FUNCTION_BLOCK "FB_ALE 203"
TITLE =
VERSION : 0.1


VAR
  WaterTemp_A1 : "fb_AnalogIN"; //Water Temperature ALE 203
WaterFlow_A1 : "fb_AnalogIN"; //Water Flowrate ALE 203
WaterTemp_A2 : "fb_AnalogIN"; //Water Temperature ALE 203
WaterFlow_A2 : "fb_AnalogIN"; //Water Flowrate ALE 203
END_VAR
BEGIN
NETWORK
TITLE =
CALL #WaterTemp_A1 (In_V_CAMPO:= PEW 316);
CALL #WaterFlow_A1 (In_V_CAMPO:= PEW 318);
CALL #WaterTemp_A2 (In_V_CAMPO:= PEW 444);
CALL #WaterFlow_A2 (In_V_CAMPO:= PEW 446);

END_FUNCTION_BLOCK

FUNCTION_BLOCK "FB_ARC_DET"
TITLE =
VERSION : 0.1


VAR
 Arc1_A1 : "fb_DI_IN"; //Water Flowrate ALE 203
PwrFail1_A1 : "fb_DI_IN"; // Arc Detector Signal 1
Arc2_A1 : "fb_DI_IN"; //Power Fail in Arc Detector 1
PwrFail2_A1 : "fb_DI_IN"; // Arc Detector Signal 2
Arc3_A1 : "fb_DI_IN"; //Power Fail in Arc Detector 2
PwrFail3_A1 : "fb_DI_IN"; // Arc Detector Signal 3
Arc4_A1 : "fb_DI_IN"; //Power Fail in Arc Detector 3
PwrFail4_A1 : "fb_DI_IN"; // Arc Detector Signal 4
Arc5_A1 : "fb_DI_IN"; //Power Fail in Arc Detector 4
PwrFail5_A1 : "fb_DI_IN"; // Arc Detector Signal 5
Arc6_A1 : "fb_DI_IN"; //Power Fail in Arc Detector 5
PwrFail6_A1 : "fb_DI_IN"; // Arc Detector Signal 6
Arc7_A1 : "fb_DI_IN"; //Power Fail in Arc Detector 6
PwrFail7_A1 : "fb_DI_IN"; // Arc Detector Signal 7
Arc8_A1 : "fb_DI_IN"; //Power Fail in Arc Detector 7
PwrFail8_A1 : "fb_DI_IN"; // Arc Detector Signal 8
Arc1_A2 : "fb_DI_IN"; //Power Fail in Arc Detector 8
PwrFail1_A2 : "fb_DI_IN"; // Arc Detector Signal 1
Arc2_A2 : "fb_DI_IN"; //Power Fail in Arc Detector 1
PwrFail2_A2 : "fb_DI_IN"; // Arc Detector Signal 2
Arc3_A2 : "fb_DI_IN"; //Power Fail in Arc Detector 2
PwrFail3_A2 : "fb_DI_IN"; // Arc Detector Signal 3
Arc4_A2 : "fb_DI_IN"; //Power Fail in Arc Detector 3
PwrFail4_A2 : "fb_DI_IN"; // Arc Detector Signal 4
Arc5_A2 : "fb_DI_IN"; //Power Fail in Arc Detector 4
PwrFail5_A2 : "fb_DI_IN"; // Arc Detector Signal 5
Arc6_A2 : "fb_DI_IN"; //Power Fail in Arc Detector 5
PwrFail6_A2 : "fb_DI_IN"; // Arc Detector Signal 6
Arc7_A2 : "fb_DI_IN"; //Power Fail in Arc Detector 6
PwrFail7_A2 : "fb_DI_IN"; // Arc Detector Signal 7
Arc8_A2 : "fb_DI_IN"; //Power Fail in Arc Detector 7
PwrFail8_A2 : "fb_DI_IN"; // Arc Detector Signal 8
END_VAR
BEGIN
NETWORK
TITLE =
CALL #Arc1_A1 (V_CAMPO:= E 8.1);
CALL #PwrFail1_A1 (V_CAMPO:= E 8.3);
CALL #Arc2_A1 (V_CAMPO:= E 8.5);
CALL #PwrFail2_A1 (V_CAMPO:= E 8.7);
CALL #Arc3_A1 (V_CAMPO:= E 9.1);
CALL #PwrFail3_A1 (V_CAMPO:= E 9.3);
CALL #Arc4_A1 (V_CAMPO:= E 9.5);
CALL #PwrFail4_A1 (V_CAMPO:= E 9.7);
CALL #Arc5_A1 (V_CAMPO:= E 10.3);
CALL #PwrFail5_A1 (V_CAMPO:= E 10.5);
CALL #Arc6_A1 (V_CAMPO:= E 10.7);
CALL #PwrFail6_A1 (V_CAMPO:= E 11.1);
CALL #Arc7_A1 (V_CAMPO:= E 11.3);
CALL #PwrFail7_A1 (V_CAMPO:= E 11.5);
CALL #Arc8_A1 (V_CAMPO:= E 11.7);
CALL #PwrFail8_A1 (V_CAMPO:= E 12.1);
CALL #Arc1_A2 (V_CAMPO:= E 32.1);
CALL #PwrFail1_A2 (V_CAMPO:= E 32.3);
CALL #Arc2_A2 (V_CAMPO:= E 32.5);
CALL #PwrFail2_A2 (V_CAMPO:= E 32.7);
CALL #Arc3_A2 (V_CAMPO:= E 33.1);
CALL #PwrFail3_A2 (V_CAMPO:= E 33.3);
CALL #Arc4_A2 (V_CAMPO:= E 33.5);
CALL #PwrFail4_A2 (V_CAMPO:= E 33.7);
CALL #Arc5_A2 (V_CAMPO:= E 34.3);
CALL #PwrFail5_A2 (V_CAMPO:= E 34.5);
CALL #Arc6_A2 (V_CAMPO:= E 34.7);
CALL #PwrFail6_A2 (V_CAMPO:= E 35.1);
CALL #Arc7_A2 (V_CAMPO:= E 35.3);
CALL #PwrFail7_A2 (V_CAMPO:= E 35.5);
CALL #Arc8_A2 (V_CAMPO:= E 35.7);
CALL #PwrFail8_A2 (V_CAMPO:= E 36.1);

END_FUNCTION_BLOCK

FUNCTION_BLOCK "FB_ARC_GLOB"
TITLE =
VERSION : 0.1


VAR
 Arc_A2 : "fb_AnalogIN"; //Global Arc
Arc : "fb_AnalogIN"; //Global Arc
GlobReset_AC : "fb_DI_OUT"; //Global Arc
GlobTest_AC : "fb_DI_OUT"; //Global Reset
GlobReset_A2 : "fb_DI_OUT"; //Global Test
GlobTest_A2 : "fb_DI_OUT"; //Global Reset
END_VAR
BEGIN
NETWORK
TITLE =
CALL #Arc_A2 (In_V_CAMPO:= PEW 462);
CALL #Arc (In_V_CAMPO:= PEW 334);
CALL #GlobReset_AC (OUT:= A 16.0);
CALL #GlobTest_AC (OUT:= A 16.1);
CALL #GlobReset_A2 (OUT:= A 32.0);
CALL #GlobTest_A2 (OUT:= A 32.1);

END_FUNCTION_BLOCK
FUNCTION_BLOCK "FB_CIRC"
TITLE =
VERSION : 0.1


VAR
 Arc_A2 : "fb_AnalogIN"; //Global Arc
Arc : "fb_AnalogIN"; //Global Arc
GlobReset_AC : "fb_DI_OUT"; //Global Arc
GlobTest_AC : "fb_DI_OUT"; //Global Reset
GlobReset_A2 : "fb_DI_OUT"; //Global Test
GlobTest_A2 : "fb_DI_OUT"; //Global Reset
END_VAR
BEGIN
NETWORK
TITLE =
CALL #Arc_A2 (In_V_CAMPO:= PEW 462);
CALL #Arc (In_V_CAMPO:= PEW 334);
CALL #GlobReset_AC (OUT:= A 16.0);
CALL #GlobTest_AC (OUT:= A 16.1);
CALL #GlobReset_A2 (OUT:= A 32.0);
CALL #GlobTest_A2 (OUT:= A 32.1);

END_FUNCTION_BLOCK
FUNCTION_BLOCK "FB_CPLT"
TITLE = VERSION : 0.1
VAR
WaterRes_AC : "fb_AnalogIN"; //Resistivity
WaterPress_AC : "fb_AnalogIN"; //Pressure Input
WaterTemp_AC : "fb_AnalogIN"; //Temperature Input
END_VAR
BEGIN
NETWORK
TITLE =
CALL #WaterRes_AC (In_V_CAMPO:= PEW 288);
CALL #WaterPress_AC (In_V_CAMPO:= PEW 290);
CALL #WaterTemp_AC (In_V_CAMPO:= PEW 292);
END_FUNCTION_BLOCK
FUNCTION_BLOCK "FB_CSPS"
 TITLE =
 VERSION : 0.1
 VAR
Vread1_1_A1 : "fb_AnalogIN"; //Voltage Monitor 1.1
Vread1_2_A1 : "fb_AnalogIN"; //Voltage Monitor 1.2
Vread1_3_A1 : "fb_AnalogIN"; //Voltage Monitor 1.3
Vread1_4_A1 : "fb_AnalogIN"; //Voltage Monitor 1.4
Vread1_1_A2 : "fb_AnalogIN"; //Voltage Monitor 2.1
Vread1_2_A2 : "fb_AnalogIN"; //Voltage Monitor 2.2
Vread1_3_A2 : "fb_AnalogIN"; //Voltage Monitor 2.3
Vread1_4_A2 : "fb_AnalogIN"; //Voltage Monitor 2.4
END_VAR
BEGIN
NETWORK
TITLE =
CALL #Vread1_1_A1 (In_V_CAMPO:= PEW 352);
CALL #Vread1_2_A1 (In_V_CAMPO:= PEW 354);
CALL #Vread1_3_A1 (In_V_CAMPO:= PEW 356);
CALL #Vread1_4_A1 (In_V_CAMPO:= PEW 358);
CALL #Vread1_1_A2 (In_V_CAMPO:= PEW 480);
CALL #Vread1_2_A2 (In_V_CAMPO:= PEW 482);
CALL #Vread1_3_A2 (In_V_CAMPO:= PEW 484);
CALL #Vread1_4_A2 (In_V_CAMPO:= PEW 486);

END_FUNCTION_BLOCK
FUNCTION_BLOCK "FB_DAMP_ACSI"
TITLE =
VERSION : 0.1 VAR
AirPress_A1 : "fb_AnalogIN"; //TH561 Air Press (RF Input)
AirPress_A2 : "fb_AnalogIN"; //TH561 Air Press (RF Input)
AirFlow_A1 : "fb_DI_IN"; //TH561 Air Press (RF Input)
AirFlow_A2 : "fb_DI_IN"; //TH561 Air Flow-rate (RF Input)

END_VAR BEGIN NETWORK TITLE =
CALL #AirPress_A1 (In_V_CAMPO:= PEW 268);
CALL #AirPress_A2 (In_V_CAMPO:= PEW 396);
CALL #AirFlow_A1 (V_CAMPO:= E 16.4);
CALL #AirFlow_A2 (V_CAMPO:= E 40.4);
END_FUNCTION_BLOCK
 FUNCTION_BLOCK "FB_DAMP_ACSO"
TITLE = VERSION : 0.1
VAR
AirPress_A1 : "fb_AnalogIN"; //TH561 Air Press (RF Output)
AirPress_A2 : "fb_AnalogIN"; //TH561 Air Press (RF Output)
AirFlow_A1 : "fb_DI_IN"; //TH561 Air Press (RF Output)
AirFlow_A2 : "fb_DI_IN"; //TH561 Air Flow-rate (RF Output)
END_VAR
BEGIN
NETWORK
TITLE =
CALL #AirPress_A1 (In_V_CAMPO:= PEW 270);
CALL #AirPress_A2 (In_V_CAMPO:= PEW 398);
CALL #AirFlow_A1 (V_CAMPO:= E 16.6);
CALL #AirFlow_A2 (V_CAMPO:= E 40.6);
END_FUNCTION_BLOCK
 FUNCTION_BLOCK "FB_DAMP_ANOD"
TITLE = VERSION : 0.1
VAR
WaterTemp_A1 : "fb_AnalogIN"; //Anode Temperature Output
WaterFlow_A1 : "fb_AnalogIN"; //Anode water Flowrate
WaterTemp_A2 : "fb_AnalogIN"; //Anode Temperature Output
WaterFlow_A2 : "fb_AnalogIN"; //Anode water Flowrate

END_VAR
BEGIN
NETWORK
TITLE =
CALL #WaterTemp_A1 (In_V_CAMPO:= PEW 304);
CALL #WaterFlow_A1 (In_V_CAMPO:= PEW 306);
CALL #WaterTemp_A2 (In_V_CAMPO:= PEW 432);
CALL #WaterFlow_A2 (In_V_CAMPO:= PEW 434);
END_FUNCTION_BLOCK
 FUNCTION_BLOCK "FB_DAMP_ANPS"
TITLE = VERSION : 0.1
VAR
Vread_A1 : "fb_AnalogIN"; //Voltage Meter
Iread_A1 : "fb_AnalogIN"; //Current Meter
Vanalog_A1 : "fb_AnalogIN"; //Charging voltage waveform
Vread_A2 : "fb_AnalogIN"; //Voltage Meter
Iread_A2 : "fb_AnalogIN"; //Current Meter
Vanalog_A2 : "fb_AnalogIN"; //Charging voltage waveform
Vset_A1 : "fb_AnalogOut"; //Charging voltage waveform
Adwellin_A1 : "fb_AnalogOut"; //Vout Voltage Programming
Vset_A2 : "fb_AnalogOut"; //Auto Dwell
Adwellin_A2 : "fb_AnalogOut"; //Vout Voltage Programming
Enable_A1 : "fb_DI_OUT"; //Auto Dwell
Inhibit_A1 : "fb_DI_OUT"; //ON/OFF
EXT_INTERLOOK_A1 : "fb_DI_OUT"; //INHIBIT
EXT_POWER_A1 : "fb_DI_OUT"; //Ext_InterLook
Enable_A2 : "fb_DI_OUT"; //Ext_Power
Inhibit_A2 : "fb_DI_OUT"; //ON/OFF
EXT_INTERLOOK_A2 : "fb_DI_OUT"; //INHIBIT
EXT_POWER_A2 : "fb_DI_OUT"; //Ext_InterLook
Ready_A1 : "fb_DI_IN"; //Ext_Power
InhibitRtn_A1 : "fb_DI_IN"; //Ready
EndOfChrge_A1 : "fb_DI_IN"; //INHIBIT
ExcRevers_A1 : "fb_DI_IN"; //End of Charge
CoolantWrn_A1 : "fb_DI_IN"; //Excess Reversal
Overvolt_A1 : "fb_DI_IN"; //Coolant Warning
Arc_A1 : "fb_DI_IN"; //Over Voltage
Interlock_A1 : "fb_DI_IN"; //ARC
InFault_A1 : "fb_DI_IN"; //Interlock
AdwellOut_A1 : "fb_DI_IN"; //Input Power Fault
LoadFault_A1 : "fb_DI_IN"; //Auto Dwell Output
CoolantFlt_A1 : "fb_DI_IN"; //Load Fault
PurgePump_A1 : "fb_DI_IN"; //Coolant Fault
Ready_A2 : "fb_DI_IN"; //Purge Pump
InhibitRtn_A2 : "fb_DI_IN"; //Ready
EndOfChrge_A2 : "fb_DI_IN"; //INHIBIT
ExcRevers_A2 : "fb_DI_IN"; //End of Charge
CoolantWrn_A2 : "fb_DI_IN"; //Excess Reversal
Overvolt_A2 : "fb_DI_IN"; //Coolant Warning
Arc_A2 : "fb_DI_IN"; //Over Voltage
Interlock_A2 : "fb_DI_IN"; //ARC
InFault_A2 : "fb_DI_IN"; //Interlock
AdwellOut_A2 : "fb_DI_IN"; //Input Power Fault
LoadFault_A2 : "fb_DI_IN"; //Auto Dwell Output
CoolantFlt_A2 : "fb_DI_IN"; //Load Fault
PurgePump_A2 : "fb_DI_IN"; //Coolant Fault
END_VAR
BEGIN
NETWORK
TITLE =
CALL #Vread_A1 (In_V_CAMPO:= PEW 360);
CALL #Iread_A1 (In_V_CAMPO:= PEW 362);
CALL #Vanalog_A1 (In_V_CAMPO:= PEW 364);
CALL #Vread_A2 (In_V_CAMPO:= PEW 488);
CALL #Iread_A2 (In_V_CAMPO:= PEW 490);
CALL #Vanalog_A2 (In_V_CAMPO:= PEW 492);
CALL #Vset_A1 (PAW_OUT:= PAW 272);
CALL #Adwellin_A1 (PAW_OUT:= PAW 274);
CALL #Vset_A2 (PAW_OUT:= PAW 304);
CALL #Adwellin_A2 (PAW_OUT:= PAW 306);
CALL #Enable_A1 (OUT:= A 24.0);
CALL #Inhibit_A1 (OUT:= A 24.1);
CALL #EXT_INTERLOOK_A1 (OUT:= A 24.2);
CALL #EXT_POWER_A1 (OUT:= A 24.3);
CALL #Enable_A2 (OUT:= A 36.0);
CALL #Inhibit_A2 (OUT:= A 36.1);
CALL #EXT_INTERLOOK_A2 (OUT:= A 36.2);
CALL #EXT_POWER_A2 (OUT:= A 36.3);
CALL #Ready_A1 (V_CAMPO:= E 12.3);
CALL #InhibitRtn_A1 (V_CAMPO:= E 12.5);
CALL #EndOfChrge_A1 (V_CAMPO:= E 12.7);
CALL #ExcRevers_A1 (V_CAMPO:= E 13.1);
CALL #CoolantWrn_A1 (V_CAMPO:= E 13.3);
CALL #Overvolt_A1 (V_CAMPO:= E 13.5);
CALL #Arc_A1 (V_CAMPO:= E 13.7);
CALL #Interlock_A1 (V_CAMPO:= E 14.1);
CALL #InFault_A1 (V_CAMPO:= E 14.5);
CALL #AdwellOut_A1 (V_CAMPO:= E 14.7);
CALL #LoadFault_A1 (V_CAMPO:= E 15.1);
CALL #CoolantFlt_A1 (V_CAMPO:= E 15.3);
CALL #PurgePump_A1 (V_CAMPO:= E 15.5);
CALL #Ready_A2 (V_CAMPO:= E 36.3);
CALL #InhibitRtn_A2 (V_CAMPO:= E 36.5);
CALL #EndOfChrge_A2 (V_CAMPO:= E 36.7);
CALL #ExcRevers_A2 (V_CAMPO:= E 37.1);
CALL #CoolantWrn_A2 (V_CAMPO:= E 37.3);
CALL #Overvolt_A2 (V_CAMPO:= E 37.5);
CALL #Arc_A2 (V_CAMPO:= E 37.7);
CALL #Interlock_A2 (V_CAMPO:= E 38.1);
CALL #InFault_A2 (V_CAMPO:= E 38.5);
CALL #AdwellOut_A2 (V_CAMPO:= E 38.7);
CALL #LoadFault_A2 (V_CAMPO:= E 39.1);
CALL #CoolantFlt_A2 (V_CAMPO:= E 39.3);
CALL #PurgePump_A2 (V_CAMPO:= E 39.5);
END_FUNCTION_BLOCK
 FUNCTION_BLOCK "FB_DAMP_CAV"
TITLE = VERSION : 0.1
VAR
State_A1 : "fb_DI_IN"; //Purge Pump
State_A2 : "fb_DI_IN"; //Driver Amplifier Cavity: Open\Closed
END_VAR
BEGIN
NETWORK
TITLE =
CALL #State_A1 (V_CAMPO:= E 10.4);
CALL #State_A2 (V_CAMPO:= E 34.4);
END_FUNCTION_BLOCK

 FUNCTION_BLOCK "FB_DAMP_CGPS"
TITLE = VERSION : 0.1
VAR
Iread_A1 : "fb_AnalogIN"; //Curret Monitor
Vread_A1 : "fb_AnalogIN"; //Voltage Monitor
Status_A1 : "fb_AnalogIN"; //Power Supply OK Signal
Iread_A2 : "fb_AnalogIN"; //Curret Monitor
Vread_A2 : "fb_AnalogIN"; //Voltage Monitor
Status_A2 : "fb_AnalogIN"; //Power Supply OK Signal
Vset_A1 : "fb_AnalogOut"; //Power Supply OK Signal
Vset_A2 : "fb_AnalogOut"; //Vout Voltage Programming
Enable_A1 : "fb_DI_OUT"; //Vout Voltage Programming
Activate_A1 : "fb_DI_OUT"; //Enable/Disable
Enable_A2 : "fb_DI_OUT"; //ON/OFF
Activate_A2 : "fb_DI_OUT"; //Enable/Disable
END_VAR
BEGIN
NETWORK
TITLE =
CALL #Iread_A1 (In_V_CAMPO:= PEW 262);
CALL #Vread_A1 (In_V_CAMPO:= PEW 264);
CALL #Status_A1 (In_V_CAMPO:= PEW 266);
CALL #Iread_A2 (In_V_CAMPO:= PEW 390);
CALL #Vread_A2 (In_V_CAMPO:= PEW 392);
CALL #Status_A2 (In_V_CAMPO:= PEW 394);
CALL #Vset_A1 (PAW_OUT:= PAW 258);
CALL #Vset_A2 (PAW_OUT:= PAW 290);
CALL #Enable_A1 (OUT:= A 16.4);
CALL #Activate_A1 (OUT:= A 16.5);
CALL #Enable_A2 (OUT:= A 32.4);
CALL #Activate_A2 (OUT:= A 32.5);
END_FUNCTION_BLOCK
 FUNCTION_BLOCK "FB_DAMP_FPS"
TITLE = VERSION : 0.1
VAR
Iread_A1 : "fb_AnalogIN"; //Curret Monitor
Vread_A1 : "fb_AnalogIN"; //Voltage Monitor
Status_A1 : "fb_AnalogIN"; //Power Supply OK Signal
Iread_A2 : "fb_AnalogIN"; //Curret Monitor
Vread_A2 : "fb_AnalogIN"; //Voltage Monitor
Status_A2 : "fb_AnalogIN"; //Power Supply OK Signal
Vset_A1 : "fb_AnalogOut"; //Power Supply OK Signal
Vset_A2 : "fb_AnalogOut"; //Vout Voltage Programming
Enable_A1 : "fb_DI_OUT"; //Vout Voltage Programming
Activate_A1 : "fb_DI_OUT"; //Enable/Disable
Enable_A2 : "fb_DI_OUT"; //ON/OFF
Activate_A2 : "fb_DI_OUT"; //Enable/Disable
END_VAR
BEGIN
NETWORK
TITLE =
CALL #Iread_A1 (In_V_CAMPO:= PEW 256);
CALL #Vread_A1 (In_V_CAMPO:= PEW 258);
CALL #Status_A1 (In_V_CAMPO:= PEW 260);
CALL #Iread_A2 (In_V_CAMPO:= PEW 384);
CALL #Vread_A2 (In_V_CAMPO:= PEW 386);
CALL #Status_A2 (In_V_CAMPO:= PEW 388);
CALL #Vset_A1 (PAW_OUT:= PAW 256);
CALL #Vset_A2 (PAW_OUT:= PAW 288);
CALL #Enable_A1 (OUT:= A 16.2);
CALL #Activate_A1 (OUT:= A 16.3);
CALL #Enable_A2 (OUT:= A 32.2);
CALL #Activate_A2 (OUT:= A 32.3);
END_FUNCTION_BLOCK
 FUNCTION_BLOCK "FB_DAMP_SGPS"
TITLE = VERSION : 0.1
VAR
Iread_A1 : "fb_AnalogIN"; //Curret Monitor
Vread_A1 : "fb_AnalogIN"; //Voltage Monitor
Status_A1 : "fb_AnalogIN"; //Power Supply OK Signal
Iread_A2 : "fb_AnalogIN"; //Curret Monitor
Vread_A2 : "fb_AnalogIN"; //Voltage Monitor
Status_A2 : "fb_AnalogIN"; //Power Supply OK Signal
Vset_A1 : "fb_AnalogOut"; //Power Supply OK Signal
Vset_A2 : "fb_AnalogOut"; //Vout Voltage Programming
Enable_A1 : "fb_DI_OUT"; //Vout Voltage Programming
Activate_A1 : "fb_DI_OUT"; //Enable/Disable
Enable_A2 : "fb_DI_OUT"; //ON/OFF
Activate_A2 : "fb_DI_OUT"; //Enable/Disable
END_VAR
BEGIN
NETWORK
TITLE =
CALL #Iread_A1 (In_V_CAMPO:= PEW 272);
CALL #Vread_A1 (In_V_CAMPO:= PEW 274);
CALL #Status_A1 (In_V_CAMPO:= PEW 276);
CALL #Iread_A2 (In_V_CAMPO:= PEW 400);
CALL #Vread_A2 (In_V_CAMPO:= PEW 402);
CALL #Status_A2 (In_V_CAMPO:= PEW 404);
CALL #Vset_A1 (PAW_OUT:= PAW 260);
CALL #Vset_A2 (PAW_OUT:= PAW 292);
CALL #Enable_A1 (OUT:= A 16.6);
CALL #Activate_A1 (OUT:= A 16.7);
CALL #Enable_A2 (OUT:= A 32.6);
CALL #Activate_A2 (OUT:= A 32.7);
END_FUNCTION_BLOCK
 FUNCTION_BLOCK "FB_FAMP_ACS"
TITLE = VERSION : 0.1
VAR
AirPress_A2 : "fb_AnalogIN"; //TH781 Air Press
AirPress_A1 : "fb_AnalogIN"; //TH781 Air Press
AirFlow_A1 : "fb_DI_IN"; //TH781 Air Press
AirFlow_A2 : "fb_DI_IN"; //TH781 Air Flow Rate

END_VAR
BEGIN
NETWORK
TITLE =
CALL #AirPress_A2 (In_V_CAMPO:= PEW 460);
CALL #AirPress_A1 (In_V_CAMPO:= PEW 332);
CALL #AirFlow_A1 (V_CAMPO:= E 17.0);
CALL #AirFlow_A2 (V_CAMPO:= E 41.0);

END_FUNCTION_BLOCK
 FUNCTION_BLOCK "FB_FAMP_ANOD"
TITLE = VERSION : 0.1
VAR
WaterTemp_A2 : "fb_AnalogIN"; //Anode Temperature Output
WaterFlow_A2 : "fb_AnalogIN"; //Anode water Flowrate
WaterTemp_A1 : "fb_AnalogIN"; //Anode Temperature Output
WaterFlow_A1 : "fb_AnalogIN"; //Anode water Flowrate
END_VAR
BEGIN
NETWORK
TITLE =
CALL #WaterTemp_A2 (In_V_CAMPO:= PEW 448);
CALL #WaterFlow_A2 (In_V_CAMPO:= PEW 450);
CALL #WaterTemp_A1 (In_V_CAMPO:= PEW 320);
CALL #WaterFlow_A1 (In_V_CAMPO:= PEW 322);
END_FUNCTION_BLOCK
 FUNCTION_BLOCK "FB_FAMP_ANPS"
TITLE = VERSION : 0.1
VAR
Vread_A1 : "fb_AnalogIN"; //Voltage Meter
Iread_A1 : "fb_AnalogIN"; //Current Meter
Vanalog_A1 : "fb_AnalogIN"; //Charging voltage waveform
Vread_A2 : "fb_AnalogIN"; //Voltage Meter
Iread_A2 : "fb_AnalogIN"; //Current Meter
Vanalog_A2 : "fb_AnalogIN"; //Charging voltage waveform
Vset_A1 : "fb_AnalogOut"; //Charging voltage waveform
Adwellin_A1 : "fb_AnalogOut"; //Vout Voltage Programming
Vset_A2 : "fb_AnalogOut"; //Auto Dwell
Adwellin_A2 : "fb_AnalogOut"; //Vout Voltage Programming
Enable_A1 : "fb_DI_OUT"; //Auto Dwell
Inhibit_A1 : "fb_DI_OUT"; //ON/OFF
EXT_INTERLOOK_A1 : "fb_DI_OUT"; //INHIBIT
EXT_POWER_A1 : "fb_DI_OUT"; //Ext_InterLook
Enable_A2 : "fb_DI_OUT"; //Ext_Power
Inhibit_A2 : "fb_DI_OUT"; //ON/OFF
EXT_INTERLOOK_A2 : "fb_DI_OUT"; //INHIBIT
EXT_POWER_A2 : "fb_DI_OUT"; //Ext_InterLook
Ready_A1 : "fb_DI_IN"; //Ext_Power
InhibitRtn_A1 : "fb_DI_IN"; //Ready
EndOfChrge_A1 : "fb_DI_IN"; //INHIBIT
ExcRevers_A1 : "fb_DI_IN"; //End of Charge
CoolantWrn_A1 : "fb_DI_IN"; //Excess Reversal
Overvolt_A1 : "fb_DI_IN"; //Coolant Warning
Arc_A1 : "fb_DI_IN"; //Over Voltage
Interlock_A1 : "fb_DI_IN"; //ARC
InFault_A1 : "fb_DI_IN"; //Interlock
AdwellOut_A1 : "fb_DI_IN"; //Input Power Fault
LoadFault_A1 : "fb_DI_IN"; //Auto Dwell Output
CoolantFlt_A1 : "fb_DI_IN"; //Load Fault
PurgePump_A1 : "fb_DI_IN"; //Coolant Fault
Ready_A2 : "fb_DI_IN"; //Purge Pump
InhibitRtn_A2 : "fb_DI_IN"; //Ready
EndOfChrge_A2 : "fb_DI_IN"; //INHIBIT
ExcRevers_A2 : "fb_DI_IN"; //End of Charge
CoolantWrn_A2 : "fb_DI_IN"; //Excess Reversal
Overvolt_A2 : "fb_DI_IN"; //Coolant Warning
Arc_A2 : "fb_DI_IN"; //Over Voltage
Interlock_A2 : "fb_DI_IN"; //ARC
InFault_A2 : "fb_DI_IN"; //Interlock
AdwellOut_A2 : "fb_DI_IN"; //Input Power Fault
LoadFault_A2 : "fb_DI_IN"; //Auto Dwell Output
CoolantFlt_A2 : "fb_DI_IN"; //Load Fault
PurgePump_A2 : "fb_DI_IN"; //Coolant Fault
END_VAR
BEGIN
NETWORK
TITLE =
CALL #Vread_A1 (In_V_CAMPO:= PEW 368);
CALL #Iread_A1 (In_V_CAMPO:= PEW 370);
CALL #Vanalog_A1 (In_V_CAMPO:= PEW 372);
CALL #Vread_A2 (In_V_CAMPO:= PEW 496);
CALL #Iread_A2 (In_V_CAMPO:= PEW 498);
CALL #Vanalog_A2 (In_V_CAMPO:= PEW 500);
CALL #Vset_A1 (PAW_OUT:= PAW 276);
CALL #Adwellin_A1 (PAW_OUT:= PAW 278);
CALL #Vset_A2 (PAW_OUT:= PAW 308);
CALL #Adwellin_A2 (PAW_OUT:= PAW 310);
CALL #Enable_A1 (OUT:= A 24.4);
CALL #Inhibit_A1 (OUT:= A 24.5);
CALL #EXT_INTERLOOK_A1 (OUT:= A 24.6);
CALL #EXT_POWER_A1 (OUT:= A 24.7);
CALL #Enable_A2 (OUT:= A 36.4);
CALL #Inhibit_A2 (OUT:= A 36.5);
CALL #EXT_INTERLOOK_A2 (OUT:= A 36.6);
CALL #EXT_POWER_A2 (OUT:= A 36.7);
CALL #Ready_A1 (V_CAMPO:= E 12.2);
CALL #InhibitRtn_A1 (V_CAMPO:= E 12.4);
CALL #EndOfChrge_A1 (V_CAMPO:= E 12.6);
CALL #ExcRevers_A1 (V_CAMPO:= E 13.0);
CALL #CoolantWrn_A1 (V_CAMPO:= E 13.2);
CALL #Overvolt_A1 (V_CAMPO:= E 13.4);
CALL #Arc_A1 (V_CAMPO:= E 13.6);
CALL #Interlock_A1 (V_CAMPO:= E 14.0);
CALL #InFault_A1 (V_CAMPO:= E 14.4);
CALL #AdwellOut_A1 (V_CAMPO:= E 14.6);
CALL #LoadFault_A1 (V_CAMPO:= E 15.0);
CALL #CoolantFlt_A1 (V_CAMPO:= E 15.2);
CALL #PurgePump_A1 (V_CAMPO:= E 15.4);
CALL #Ready_A2 (V_CAMPO:= E 36.2);
CALL #InhibitRtn_A2 (V_CAMPO:= E 36.4);
CALL #EndOfChrge_A2 (V_CAMPO:= E 36.6);
CALL #ExcRevers_A2 (V_CAMPO:= E 37.0);
CALL #CoolantWrn_A2 (V_CAMPO:= E 37.2);
CALL #Overvolt_A2 (V_CAMPO:= E 37.4);
CALL #Arc_A2 (V_CAMPO:= E 37.6);
CALL #Interlock_A2 (V_CAMPO:= E 38.0);
CALL #InFault_A2 (V_CAMPO:= E 38.4);
CALL #AdwellOut_A2 (V_CAMPO:= E 38.6);
CALL #LoadFault_A2 (V_CAMPO:= E 39.0);
CALL #CoolantFlt_A2 (V_CAMPO:= E 39.2);
CALL #PurgePump_A2 (V_CAMPO:= E 39.4);
END_FUNCTION_BLOCK
 FUNCTION_BLOCK "FB_FAMP_CAV"
TITLE = VERSION : 0.1
VAR
WaterTemp_A2 : "fb_AnalogIN"; //Cavity Temperature Output
WaterFlow_A2 : "fb_AnalogIN"; //Cavity water Flowrate
WaterTemp_A1 : "fb_AnalogIN"; //Cavity Temperature Output
WaterFlow_A1 : "fb_AnalogIN"; //Cavity water Flowrate
TempInt_A1 : "fb_DI_IN"; //Cavity water Flowrate
TempInt_A2 : "fb_DI_IN"; //F A Cavity: Temperature Switch
END_VAR
BEGIN
NETWORK
TITLE =
CALL #WaterTemp_A2 (In_V_CAMPO:= PEW 456);
CALL #WaterFlow_A2 (In_V_CAMPO:= PEW 458);
CALL #WaterTemp_A1 (In_V_CAMPO:= PEW 328);
CALL #WaterFlow_A1 (In_V_CAMPO:= PEW 330);
CALL #TempInt_A1 (V_CAMPO:= E 10.6);
CALL #TempInt_A2 (V_CAMPO:= E 34.6);
END_FUNCTION_BLOCK
 FUNCTION_BLOCK "FB_FAMP_CGPS"
TITLE = VERSION : 0.1
VAR
Iread_A1 : "fb_AnalogIN"; //Curret Monitor
Vread_A1 : "fb_AnalogIN"; //Voltage Monitor
Status_A1 : "fb_AnalogIN"; //Power Supply OK Signal
Iread_A2 : "fb_AnalogIN"; //Curret Monitor
Vread_A2 : "fb_AnalogIN"; //Voltage Monitor
Status_A2 : "fb_AnalogIN"; //Power Supply OK Signal
Vset_A1 : "fb_AnalogOut"; //Power Supply OK Signal
Vset_A2 : "fb_AnalogOut"; //Vout Voltage Programming
Enable_A1 : "fb_DI_OUT"; //Vout Voltage Programming
Activate_A1 : "fb_DI_OUT"; //Enable/Disable
Enable_A2 : "fb_DI_OUT"; //ON/OFF
Activate_A2 : "fb_DI_OUT"; //Enable/Disable
END_VAR
BEGIN
NETWORK
TITLE =
CALL #Iread_A1 (In_V_CAMPO:= PEW 342);
CALL #Vread_A1 (In_V_CAMPO:= PEW 344);
CALL #Status_A1 (In_V_CAMPO:= PEW 346);
CALL #Iread_A2 (In_V_CAMPO:= PEW 470);
CALL #Vread_A2 (In_V_CAMPO:= PEW 472);
CALL #Status_A2 (In_V_CAMPO:= PEW 474);
CALL #Vset_A1 (PAW_OUT:= PAW 264);
CALL #Vset_A2 (PAW_OUT:= PAW 296);
CALL #Enable_A1 (OUT:= A 17.2);
CALL #Activate_A1 (OUT:= A 17.3);
CALL #Enable_A2 (OUT:= A 33.2);
CALL #Activate_A2 (OUT:= A 33.3);
END_FUNCTION_BLOCK
 FUNCTION_BLOCK "FB_FAMP_FPS"
TITLE = VERSION : 0.1
VAR
Iread_A1 : "fb_AnalogIN"; //Curret Monitor
Vread_A1 : "fb_AnalogIN"; //Voltage Monitor
Status_A1 : "fb_AnalogIN"; //Power Supply OK Signal
Iread_A2 : "fb_AnalogIN"; //Curret Monitor
Vread_A2 : "fb_AnalogIN"; //Voltage Monitor
Status_A2 : "fb_AnalogIN"; //Power Supply OK Signal
Vset_A1 : "fb_AnalogOut"; //Power Supply OK Signal
Vset_A2 : "fb_AnalogOut"; //Vout Voltage Programming
Activate_A1 : "fb_DI_OUT"; //Vout Voltage Programming
Enable_A1 : "fb_DI_OUT"; //ON/OFF
Activate_A2 : "fb_DI_OUT"; //Enable/Disable
Enable_A2 : "fb_DI_OUT"; //ON/OFF
END_VAR
BEGIN
NETWORK
TITLE =
CALL #Iread_A1 (In_V_CAMPO:= PEW 336);
CALL #Vread_A1 (In_V_CAMPO:= PEW 338);
CALL #Status_A1 (In_V_CAMPO:= PEW 340);
CALL #Iread_A2 (In_V_CAMPO:= PEW 464);
CALL #Vread_A2 (In_V_CAMPO:= PEW 466);
CALL #Status_A2 (In_V_CAMPO:= PEW 468);
CALL #Vset_A1 (PAW_OUT:= PAW 262);
CALL #Vset_A2 (PAW_OUT:= PAW 294);
CALL #Activate_A1 (OUT:= A 17.1);
CALL #Enable_A1 (OUT:= A 17.0);
CALL #Activate_A2 (OUT:= A 33.1);
CALL #Enable_A2 (OUT:= A 33.0);
END_FUNCTION_BLOCK
 FUNCTION_BLOCK "FB_FAMP_SCRE"
TITLE = VERSION : 0.1
VAR
WaterTemp_A2 : "fb_AnalogIN"; //Screen-grid Temperature Output
WaterFlow_A2 : "fb_AnalogIN"; //Screen-grid water Flowrate
WaterTemp_A1 : "fb_AnalogIN"; //Screen-grid Temperature Output
WaterFlow_A1 : "fb_AnalogIN"; //Screen-grid water Flowrate
END_VAR
BEGIN
NETWORK
TITLE =
CALL #WaterTemp_A2 (In_V_CAMPO:= PEW 452);
CALL #WaterFlow_A2 (In_V_CAMPO:= PEW 454);
CALL #WaterTemp_A1 (In_V_CAMPO:= PEW 324);
CALL #WaterFlow_A1 (In_V_CAMPO:= PEW 326);
END_FUNCTION_BLOCK
 FUNCTION_BLOCK "FB_FAMP_SGPS"
TITLE = VERSION : 0.1
VAR
Vread1_A1 : "fb_AnalogIN"; //Voltage Monitor
Status_A1 : "fb_AnalogIN"; //Power Supply OK Signal
Vread2_A1 : "fb_AnalogIN"; //Voltage Monitor
Vread3_A1 : "fb_AnalogIN"; //Voltage Monitor
Vread1_A2 : "fb_AnalogIN"; //Voltage Monitor
Status_A2 : "fb_AnalogIN"; //Power Supply OK Signal
Vread2_A2 : "fb_AnalogIN"; //Voltage Monitor
Vread3_A2 : "fb_AnalogIN"; //Voltage Monitor
Activate_A1 : "fb_DI_OUT"; //Voltage Monitor
Activate_A2 : "fb_DI_OUT"; //ON/OFF
END_VAR
BEGIN
NETWORK
TITLE =
CALL #Vread1_A1 (In_V_CAMPO:= PEW 280);
CALL #Status_A1 (In_V_CAMPO:= PEW 282);
CALL #Vread2_A1 (In_V_CAMPO:= PEW 284);
CALL #Vread3_A1 (In_V_CAMPO:= PEW 286);
CALL #Vread1_A2 (In_V_CAMPO:= PEW 408);
CALL #Status_A2 (In_V_CAMPO:= PEW 410);
CALL #Vread2_A2 (In_V_CAMPO:= PEW 412);
CALL #Vread3_A2 (In_V_CAMPO:= PEW 414);
CALL #Activate_A1 (OUT:= A 17.4);
CALL #Activate_A2 (OUT:= A 33.4);
END_FUNCTION_BLOCK
 FUNCTION_BLOCK "FB_FAMP_SGPS.1"
TITLE = VERSION : 0.1
VAR
Vset1_A1 : "fb_AnalogOut"; //ON/OFF
Vset1_A2 : "fb_AnalogOut"; //Vout Voltage Programming
Enable_A1 : "fb_DI_OUT"; //Vout Voltage Programming
Enable_A2 : "fb_DI_OUT"; //Enable/Disable
END_VAR
BEGIN
NETWORK
TITLE =
CALL #Vset1_A1 (PAW_OUT:= PAW 266);
CALL #Vset1_A2 (PAW_OUT:= PAW 298);
CALL #Enable_A1 (OUT:= A 17.5);
CALL #Enable_A2 (OUT:= A 33.5);
END_FUNCTION_BLOCK
 FUNCTION_BLOCK "FB_FAMP_SGPS.2"
TITLE = VERSION : 0.1
VAR
Vset2_A1 : "fb_AnalogOut"; //Enable/Disable
Vset2_A2 : "fb_AnalogOut"; //Vout Voltage Programming
Enable_A1 : "fb_DI_OUT"; //Vout Voltage Programming
Enable_A2 : "fb_DI_OUT"; //Enable/Disable
END_VAR
BEGIN
NETWORK
TITLE =
CALL #Vset2_A1 (PAW_OUT:= PAW 268);
CALL #Vset2_A2 (PAW_OUT:= PAW 300);
CALL #Enable_A1 (OUT:= A 21.4);
CALL #Enable_A2 (OUT:= A 35.4);
END_FUNCTION_BLOCK
 FUNCTION_BLOCK "FB_FAMP_SGPS.3"
TITLE = VERSION : 0.1
VAR
Vset3_A1 : "fb_AnalogOut"; //Enable/Disable
Vset3_A2 : "fb_AnalogOut"; //Vout Voltage Programming
Enable_A1 : "fb_DI_OUT"; //Vout Voltage Programming
Enable_A2 : "fb_DI_OUT"; //Enable/Disable
END_VAR
BEGIN
NETWORK
TITLE =
CALL #Vset3_A1 (PAW_OUT:= PAW 270);
CALL #Vset3_A2 (PAW_OUT:= PAW 302);
CALL #Enable_A1 (OUT:= A 21.5);
CALL #Enable_A2 (OUT:= A 35.5);
END_FUNCTION_BLOCK
 FUNCTION_BLOCK "FB_FAMP_SGPS1"
TITLE = VERSION : 0.1
VAR
Iread1_A1 : "fb_AnalogIN"; //Curret Monitor
Iread1_A2 : "fb_AnalogIN"; //Curret Monitor
END_VAR
BEGIN
NETWORK
TITLE =
CALL #Iread1_A1 (In_V_CAMPO:= PEW 278);
CALL #Iread1_A2 (In_V_CAMPO:= PEW 406);
END_FUNCTION_BLOCK
 FUNCTION_BLOCK "FB_IDENT  RRF MODULE"
TITLE = VERSION : 0.1
VAR
ModuleType_AC : "fb_DI_IN"; //Curret Monitor
END_VAR
BEGIN
NETWORK
TITLE =
CALL #ModuleType_AC (V_CAMPO:= E 12.0);
END_FUNCTION_BLOCK
 FUNCTION_BLOCK "FB_LLRF"
TITLE = VERSION : 0.1
VAR
RfDet_A1 : "fb_AnalogIN"; //RF Detector Output
RfDet_A2 : "fb_AnalogIN"; //RF Detector Output
IntOutput_A1 : "fb_AnalogOut"; //RF Detector Output
IntOutput_A2 : "fb_AnalogOut"; //Interlock Output (to LLRF)
Vaacum2_A1 : "fb_DI_OUT"; //Interlock Output (to LLRF)
Vaacum1_A1 : "fb_DI_OUT"; //DO VAACUM
Vaacum2_A2 : "fb_DI_OUT"; //DO VAACUM
Vaacum1_A2 : "fb_DI_OUT"; //DO VAACUM
IntInput_A1 : "fb_DI_IN"; //DO VAACUM
IntInput_A2 : "fb_DI_IN"; //Interlock Input (From LLRF)
END_VAR
BEGIN
NETWORK
TITLE =
CALL #RfDet_A1 (In_V_CAMPO:= PEW 366);
CALL #RfDet_A2 (In_V_CAMPO:= PEW 494);
CALL #IntOutput_A1 (PAW_OUT:= PAW 280);
CALL #IntOutput_A2 (PAW_OUT:= PAW 312);
CALL #Vaacum2_A1 (OUT:= A 25.1);
CALL #Vaacum1_A1 (OUT:= A 25.0);
CALL #Vaacum2_A2 (OUT:= A 37.1);
CALL #Vaacum1_A2 (OUT:= A 37.0);
CALL #IntInput_A1 (V_CAMPO:= E 17.2);
CALL #IntInput_A2 (V_CAMPO:= E 40.2);
END_FUNCTION_BLOCK
 FUNCTION_BLOCK "FB_LOAD"
TITLE = VERSION : 0.1
VAR
WaterTemp_A1 : "fb_AnalogIN"; //Water Temperature at Load's Output
WaterFlow_A1 : "fb_AnalogIN"; //Water Flowrate at Load's Output
WaterTemp_A2 : "fb_AnalogIN"; //Water Temperature at Load's Output
WaterFlow_A2 : "fb_AnalogIN"; //Water Flowrate at Load's Output
END_VAR
BEGIN
NETWORK
TITLE =
CALL #WaterTemp_A1 (In_V_CAMPO:= PEW 312);
CALL #WaterFlow_A1 (In_V_CAMPO:= PEW 314);
CALL #WaterTemp_A2 (In_V_CAMPO:= PEW 440);
CALL #WaterFlow_A2 (In_V_CAMPO:= PEW 442);
END_FUNCTION_BLOCK
 FUNCTION_BLOCK "FB_MPAC_DET"
TITLE = VERSION : 0.1
VAR
Multipact1_A1 : "fb_AnalogIN"; //AI Multipacting
Multipact2_A1 : "fb_AnalogIN"; //AI Multipacting
Multipact1_A2 : "fb_AnalogIN"; //AI Multipacting
Multipact2_A2 : "fb_AnalogIN"; //AI Multipacting
END_VAR
BEGIN
NETWORK
TITLE =
CALL #Multipact1_A1 (In_V_CAMPO:= PEW 294);
CALL #Multipact2_A1 (In_V_CAMPO:= PEW 296);
CALL #Multipact1_A2 (In_V_CAMPO:= PEW 416);
CALL #Multipact2_A2 (In_V_CAMPO:= PEW 418);
END_FUNCTION_BLOCK
 FUNCTION_BLOCK "FB_MPLT"
TITLE = VERSION : 0.1
VAR
AirTemp_AC : "fb_AnalogIN"; //AirTemp
BlowerCtrl_A1 : "fb_DI_OUT"; //AirTemp
END_VAR
BEGIN
NETWORK
TITLE =
CALL #AirTemp_AC (In_V_CAMPO:= PEW 374);
CALL #BlowerCtrl_A1 (OUT:= A 25.4);
END_FUNCTION_BLOCK
 FUNCTION_BLOCK "FB_MPS"
TITLE = VERSION : 0.1
VAR
Fault_A1 : "fb_DI_OUT"; //Switch On\Off Blower
Fault_A2 : "fb_DI_OUT"; //Fault Signal
END_VAR
BEGIN
NETWORK
TITLE =
CALL #Fault_A1 (OUT:= A 25.3);
CALL #Fault_A2 (OUT:= A 37.3);
END_FUNCTION_BLOCK
 FUNCTION_BLOCK "FB_PPS"
TITLE = VERSION : 0.1
VAR
Enable_A1 : "fb_DI_IN"; //Fault Signal
Enable_A2 : "fb_DI_IN"; //Power Permission Signal
END_VAR
BEGIN
NETWORK
TITLE =
CALL #Enable_A1 (V_CAMPO:= E 18.0);
CALL #Enable_A2 (V_CAMPO:= E 42.0);
END_FUNCTION_BLOCK
 FUNCTION_BLOCK "FB_PSYS"
TITLE = VERSION : 0.1
VAR
Inhibit : "fb_DI_OUT"; //Power Permission Signal
Interlock : "fb_DI_IN"; //Inhibit Protection System
END_VAR
BEGIN
NETWORK
TITLE =
CALL #Inhibit (OUT:= A 25.7);
CALL #Interlock (V_CAMPO:= E 18.2);
END_FUNCTION_BLOCK
 FUNCTION_BLOCK "FB_TCU"
TITLE = VERSION : 0.1
VAR
Booting_A1 : "fb_DI_IN"; //Interlock Protection System (OC)
Status_A1 : "fb_DI_IN"; //TCU is booting
ErrCoil_A1 : "fb_DI_IN"; //TCU OK, ready for operation
ErrTinL_A1 : "fb_DI_IN"; //Error, coil not connected
ErrTinH_A1 : "fb_DI_IN"; //Error, Tin too low
ErrAmbL_A1 : "fb_DI_IN"; //Error, Iin too high
ErrdTH_A1 : "fb_DI_IN"; //Error, Tamb too low
Booting_A2 : "fb_DI_IN"; //Error, dT too high
Status_A2 : "fb_DI_IN"; //TCU is booting
ErrCoil_A2 : "fb_DI_IN"; //TCU OK, ready for operation
ErrTinL_A2 : "fb_DI_IN"; //Error, coil not connected
ErrTinH_A2 : "fb_DI_IN"; //Error, Tin too low
ErrAmbL_A2 : "fb_DI_IN"; //Error, Iin too high
ErrdTH_A2 : "fb_DI_IN"; //Error, Tamb too low
END_VAR
BEGIN
NETWORK
TITLE =
CALL #Booting_A1 (V_CAMPO:= E 8.0);
CALL #Status_A1 (V_CAMPO:= E 8.2);
CALL #ErrCoil_A1 (V_CAMPO:= E 8.4);
CALL #ErrTinL_A1 (V_CAMPO:= E 8.6);
CALL #ErrTinH_A1 (V_CAMPO:= E 9.0);
CALL #ErrAmbL_A1 (V_CAMPO:= E 9.2);
CALL #ErrdTH_A1 (V_CAMPO:= E 9.4);
CALL #Booting_A2 (V_CAMPO:= E 32.0);
CALL #Status_A2 (V_CAMPO:= E 32.2);
CALL #ErrCoil_A2 (V_CAMPO:= E 32.4);
CALL #ErrTinL_A2 (V_CAMPO:= E 32.6);
CALL #ErrTinH_A2 (V_CAMPO:= E 33.0);
CALL #ErrAmbL_A2 (V_CAMPO:= E 33.2);
CALL #ErrdTH_A2 (V_CAMPO:= E 33.4);
END_FUNCTION_BLOCK
 FUNCTION_BLOCK "FB_UPS"
TITLE = VERSION : 0.1
VAR
R1_A1 : "fb_DI_IN"; //Error, dT too high
R2_A1 : "fb_DI_IN"; //Alarma General
R3_A1 : "fb_DI_IN"; //Red Ausente
R4_A1 : "fb_DI_IN"; //Batería Baja
R5_A1 : "fb_DI_IN"; //En By-Pass
R6_A1 : "fb_DI_IN"; //Sobrecarga
END_VAR
BEGIN
NETWORK
TITLE =
CALL #R1_A1 (V_CAMPO:= E 16.1);
CALL #R2_A1 (V_CAMPO:= E 16.3);
CALL #R3_A1 (V_CAMPO:= E 16.5);
CALL #R4_A1 (V_CAMPO:= E 16.7);
CALL #R5_A1 (V_CAMPO:= E 17.1);
CALL #R6_A1 (V_CAMPO:= E 17.3);
END_FUNCTION_BLOCK
 FUNCTION_BLOCK "FB_VAC_DET"
TITLE = VERSION : 0.1
VAR
Vaacum1_A1 : "fb_AnalogIN"; //AIVaacum
Vaacum2_A1 : "fb_AnalogIN"; //AIVaacum
Vaacum3_A1 : "fb_AnalogIN"; //AIVaacum
Vaacum1_A2 : "fb_AnalogIN"; //AIVaacum
Vaacum2_A2 : "fb_AnalogIN"; //AIVaacum
Vaacum3_A2 : "fb_AnalogIN"; //AIVaacum
END_VAR
BEGIN
NETWORK
TITLE =
CALL #Vaacum1_A1 (In_V_CAMPO:= PEW 298);
CALL #Vaacum2_A1 (In_V_CAMPO:= PEW 300);
CALL #Vaacum3_A1 (In_V_CAMPO:= PEW 302);
CALL #Vaacum1_A2 (In_V_CAMPO:= PEW 420);
CALL #Vaacum2_A2 (In_V_CAMPO:= PEW 422);
CALL #Vaacum3_A2 (In_V_CAMPO:= PEW 424);
END_FUNCTION_BLOCK
